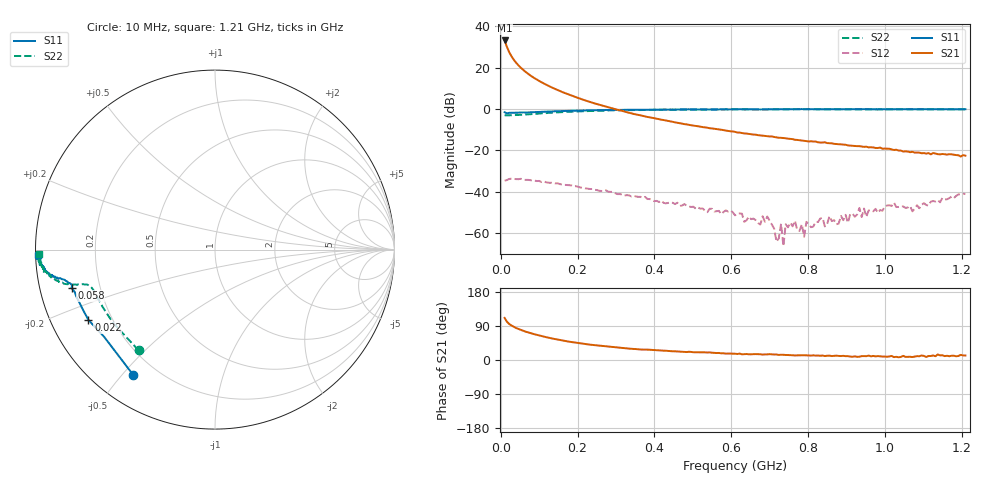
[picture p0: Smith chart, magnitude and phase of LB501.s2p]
!  POLYFET RF DEVICES
!  LB501 (Each Side)
!  S PARAMETERS
!  VDS=28V, IDQ=400mA
! Date: Thu Mar 13 09:54:24 2003
# MHZ S MA R 50
! Freq=Mhz Mag[s11] Ang[s11] Mag[s21] Ang[s21] Mag[s12] Ang[s12] Mag[s22] Ang[s22]
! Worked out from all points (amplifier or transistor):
!   201 points, 10 MHz to 1.21 GHz, reference 50 ohm
!   highest |S21| = 33.1 dB at 10 MHz (marker M1)
!   |S21| within 3 dB of that: start of sweep to 15.73 MHz
!   unconditionally stable (mu >= 1): 709 MHz to 754.2 MHz; 822.9 MHz to 930.6 MHz; 959.5 MHz to end of sweep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
!   at 208 MHz: K = 0.08, MSG = 21.5 dB, |S12| = -38.0 dB
!   at 610 MHz: K = 0.06, MSG = 20.2 dB, |S12| = -51.5 dB
!   at 1.21 GHz: K = 1.26, MAG = 6.2 dB, |S12| = -41.1 dB
!   S11 on the Smith chart (normalised r, x): 10 MHz: 0.12, -0.54; 22 MHz: 0.11, -0.26; 58 MHz: 0.10, -0.13; 1.21 GHz: 0.01, -0.01
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10  0.834 -123.1  45.45 111.0  0.01844 22.8  0.7044 -127.2
16  0.786 -141.7  31.66 101.1  0.01908 10.9  0.6996 -144.5
22  0.8068 -151.0  23.65 95.0  0.02028 6.2  0.7024 -152.5
28  0.8087 -155.9  18.78 91.0  0.02074 2.4  0.7063 -156.8
34  0.8122 -159.5  15.47 87.5  0.02042 -1.9  0.7122 -159.4
40  0.8162 -161.6  13.12 84.4  0.02009 -5.4  0.7137 -161.4
46  0.8155 -163.1  11.4 81.9  0.02 -6.4  0.7177 -162.5
58  0.8269 -165.1  8.921 77.3  0.01985 -11.4  0.7299 -164.0
82  0.8377 -167.3  6.019 69.6  0.01846 -17.3  0.7531 -165.1
112  0.8569 -168.7  4.142 61.9  0.01763 -24.4  0.7872 -165.7
160  0.8934 -170.0  2.569 51.5  0.01478 -32.6  0.8394 -166.8
214  0.9226 -171.2  1.679 42.7  0.01246 -39.4  0.8839 -168.0
412  0.9641 -174.2  0.5676 25.5  0.00561 -46.8  0.9623 -172.6
610  0.9826 -176.3  0.2795 16.6  0.00267 -24.1  0.9784 -176.0
694  0.9818 -176.3  0.2192 14.8  0.00251 18.8  0.9743 -176.7
718  0.9827 -176.6  0.2059 14.6  0.00062 -6.1  0.9819 -176.5
730  0.9795 -176.8  0.2007 13.8  0.00167 27.4  0.9817 -176.8
736  0.9835 -176.7  0.198 13.7  0.00048 15.2  0.9792 -176.7
742  0.9805 -177.0  0.1955 13.3  0.00163 11.4  0.9818 -176.9
814  0.984 -177.2  0.1632 12.4  0.00143 62.2  0.9847 -177.5
1012  0.9841 -177.5  0.1091 9.4  0.00469 94.3  0.9819 -178.2
1210  0.9868 -178.3  0.07415 11.9  0.00876 110.5  0.9804 -178.6
